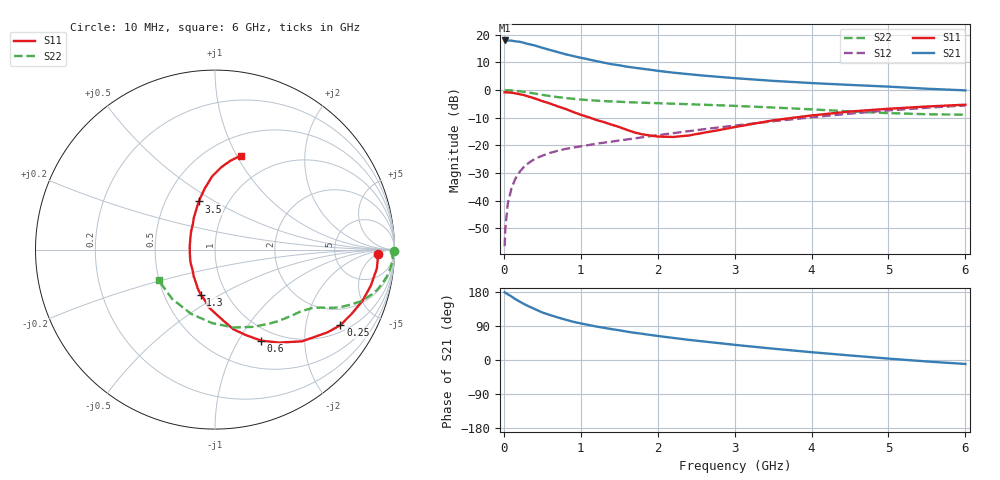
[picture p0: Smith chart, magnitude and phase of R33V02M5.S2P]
! SIEMENS Small Signal Semiconductors
! BFR181
! Si NPN RF Bipolar Junction Transistor in SOT23
! VCE = 3 V  IC = 2.5 mA
! Common Emitter S-Parameters:  May  1996
# GHz  S  MA  R  50
!  f  S11  S21  S12  S22
! GHz  MAG  ANG  MAG  ANG  MAG  ANG  MAG  ANG
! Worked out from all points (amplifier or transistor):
!   36 points, 10 MHz to 6 GHz, reference 50 ohm
!   highest |S21| = 17.9 dB at 10 MHz (marker M1)
!   |S21| within 3 dB of that: start of sweep to 543.8 MHz
!   unconditionally stable (mu >= 1): 1.479 GHz to 3.272 GHz
!   at 250 MHz: K = 0.27, MSG = 22.6 dB, |S12| = -28.1 dB
!   at 1.4 GHz: K = 0.99, MSG = 14.0 dB, |S12| = -18.7 dB
!   at 6 GHz: K = 0.86, MSG = 2.7 dB, |S12| = -5.6 dB
!   S11 on the Smith chart (normalised r, x): 10 MHz: 19, -5; 250 MHz: 1.25, -3.14; 600 MHz: 0.84, -1.25; 1.3 GHz: 0.76, -0.41; 3.5 GHz: 0.73, +0.42; 6 GHz: 0.70, +1.04
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0.01  0.9078 -1.5  7.862 178.8  0.0015 89.7  0.9958 -0.6
0.02  0.9088 -2.5  7.738 177.3  0.0032 84.3  0.9852 -1.2
0.05  0.9081 -6.6  7.854 173.7  0.0086 85.5  0.9929 -3.0
0.1  0.8909 -13.1  7.796 167.6  0.0168 83.2  0.9832 -6.0
0.15  0.8698 -19.2  7.574 160.6  0.0249 78.2  0.9694 -8.9
0.2  0.8418 -25.1  7.463 154.9  0.0322 75.4  0.951 -11.5
0.25  0.8156 -31.1  7.201 149.2  0.0393 72.0  0.9304 -14.0
0.3  0.7776 -36.4  6.872 143.9  0.0455 70.0  0.9079 -16.0
0.4  0.7046 -46.5  6.391 134.6  0.0566 65.6  0.8629 -19.5
0.5  0.6288 -55.5  5.791 125.5  0.0648 61.9  0.8156 -22.1
0.6  0.5688 -63.1  5.29 118.7  0.0728 59.7  0.776 -24.2
0.8  0.4553 -77.0  4.432 106.5  0.0859 56.6  0.7167 -26.9
0.9  0.4009 -83.0  4.108 101.0  0.091 55.9  0.693 -27.9
1.1  0.3224 -96.3  3.577 92.5  0.101 56.0  0.6551 -29.6
1.3  0.2627 -107.7  3.119 85.0  0.1116 56.1  0.6295 -31.2
1.7  0.1704 -136.9  2.527 71.8  0.1332 57.2  0.5954 -34.8
2.2  0.1415 175.4  2.059 58.3  0.1654 57.8  0.5657 -40.5
2.8  0.1886 130.8  1.725 44.5  0.2111 57.0  0.529 -49.1
3.5  0.283 108.7  1.462 29.9  0.2717 53.5  0.4824 -63.1
4.5  0.4078 92.3  1.235 12.0  0.374 44.6  0.4096 -92.4
5.5  0.5026 80.2  1.054 -3.9  0.4775 32.1  0.3642 -130.8
6  0.5421 74.7  0.984 -10.5  0.5247 24.9  0.3575 -151.6
